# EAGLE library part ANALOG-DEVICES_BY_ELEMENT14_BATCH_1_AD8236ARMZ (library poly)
40 uA Micropower Instrumentation Amplifier with Zero Crossover Distortion
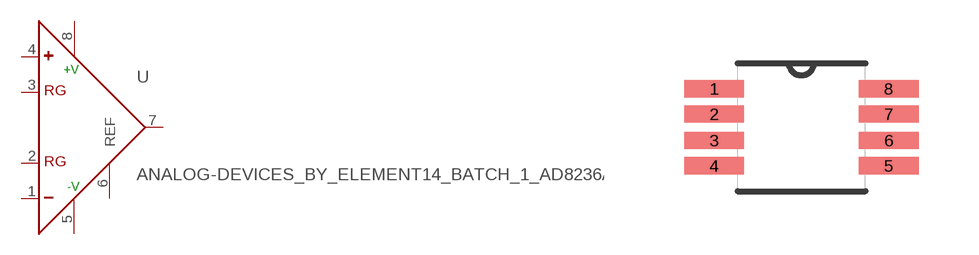
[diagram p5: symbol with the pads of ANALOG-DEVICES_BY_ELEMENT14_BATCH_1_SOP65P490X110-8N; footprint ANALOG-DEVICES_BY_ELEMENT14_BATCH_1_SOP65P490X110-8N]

Designator prefix U

## ANALOG-DEVICES_BY_ELEMENT14_BATCH_1_AD8236ARMZ (MPN: AD8236ARMZ; OC_FARNELL: 1827362; OC_NEWARK: 80R8173; PACKAGE: MSOP-8; SUPPLIER: Analog Devices)  [ANALOG-DEVICES_BY_ELEMENT14_BATCH_1_SOP65P490X110-8N]
1  -  in
2  RG  pas
3  RG  pas
4  +  in
5  -V  pwr
6  REF  pas
7  OUT  out
8  +V  pwr

## Footprint ANALOG-DEVICES_BY_ELEMENT14_BATCH_1_SOP65P490X110-8N (pad centres in mm)
smd 1.499 x 0.432: 1 -2.184,0.965; 2 -2.184,0.33; 3 -2.184,-0.33; 4 -2.184,-0.965; 5 2.184,-0.965; 6 2.184,-0.33; 7 2.184,0.33; 8 2.184,0.965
